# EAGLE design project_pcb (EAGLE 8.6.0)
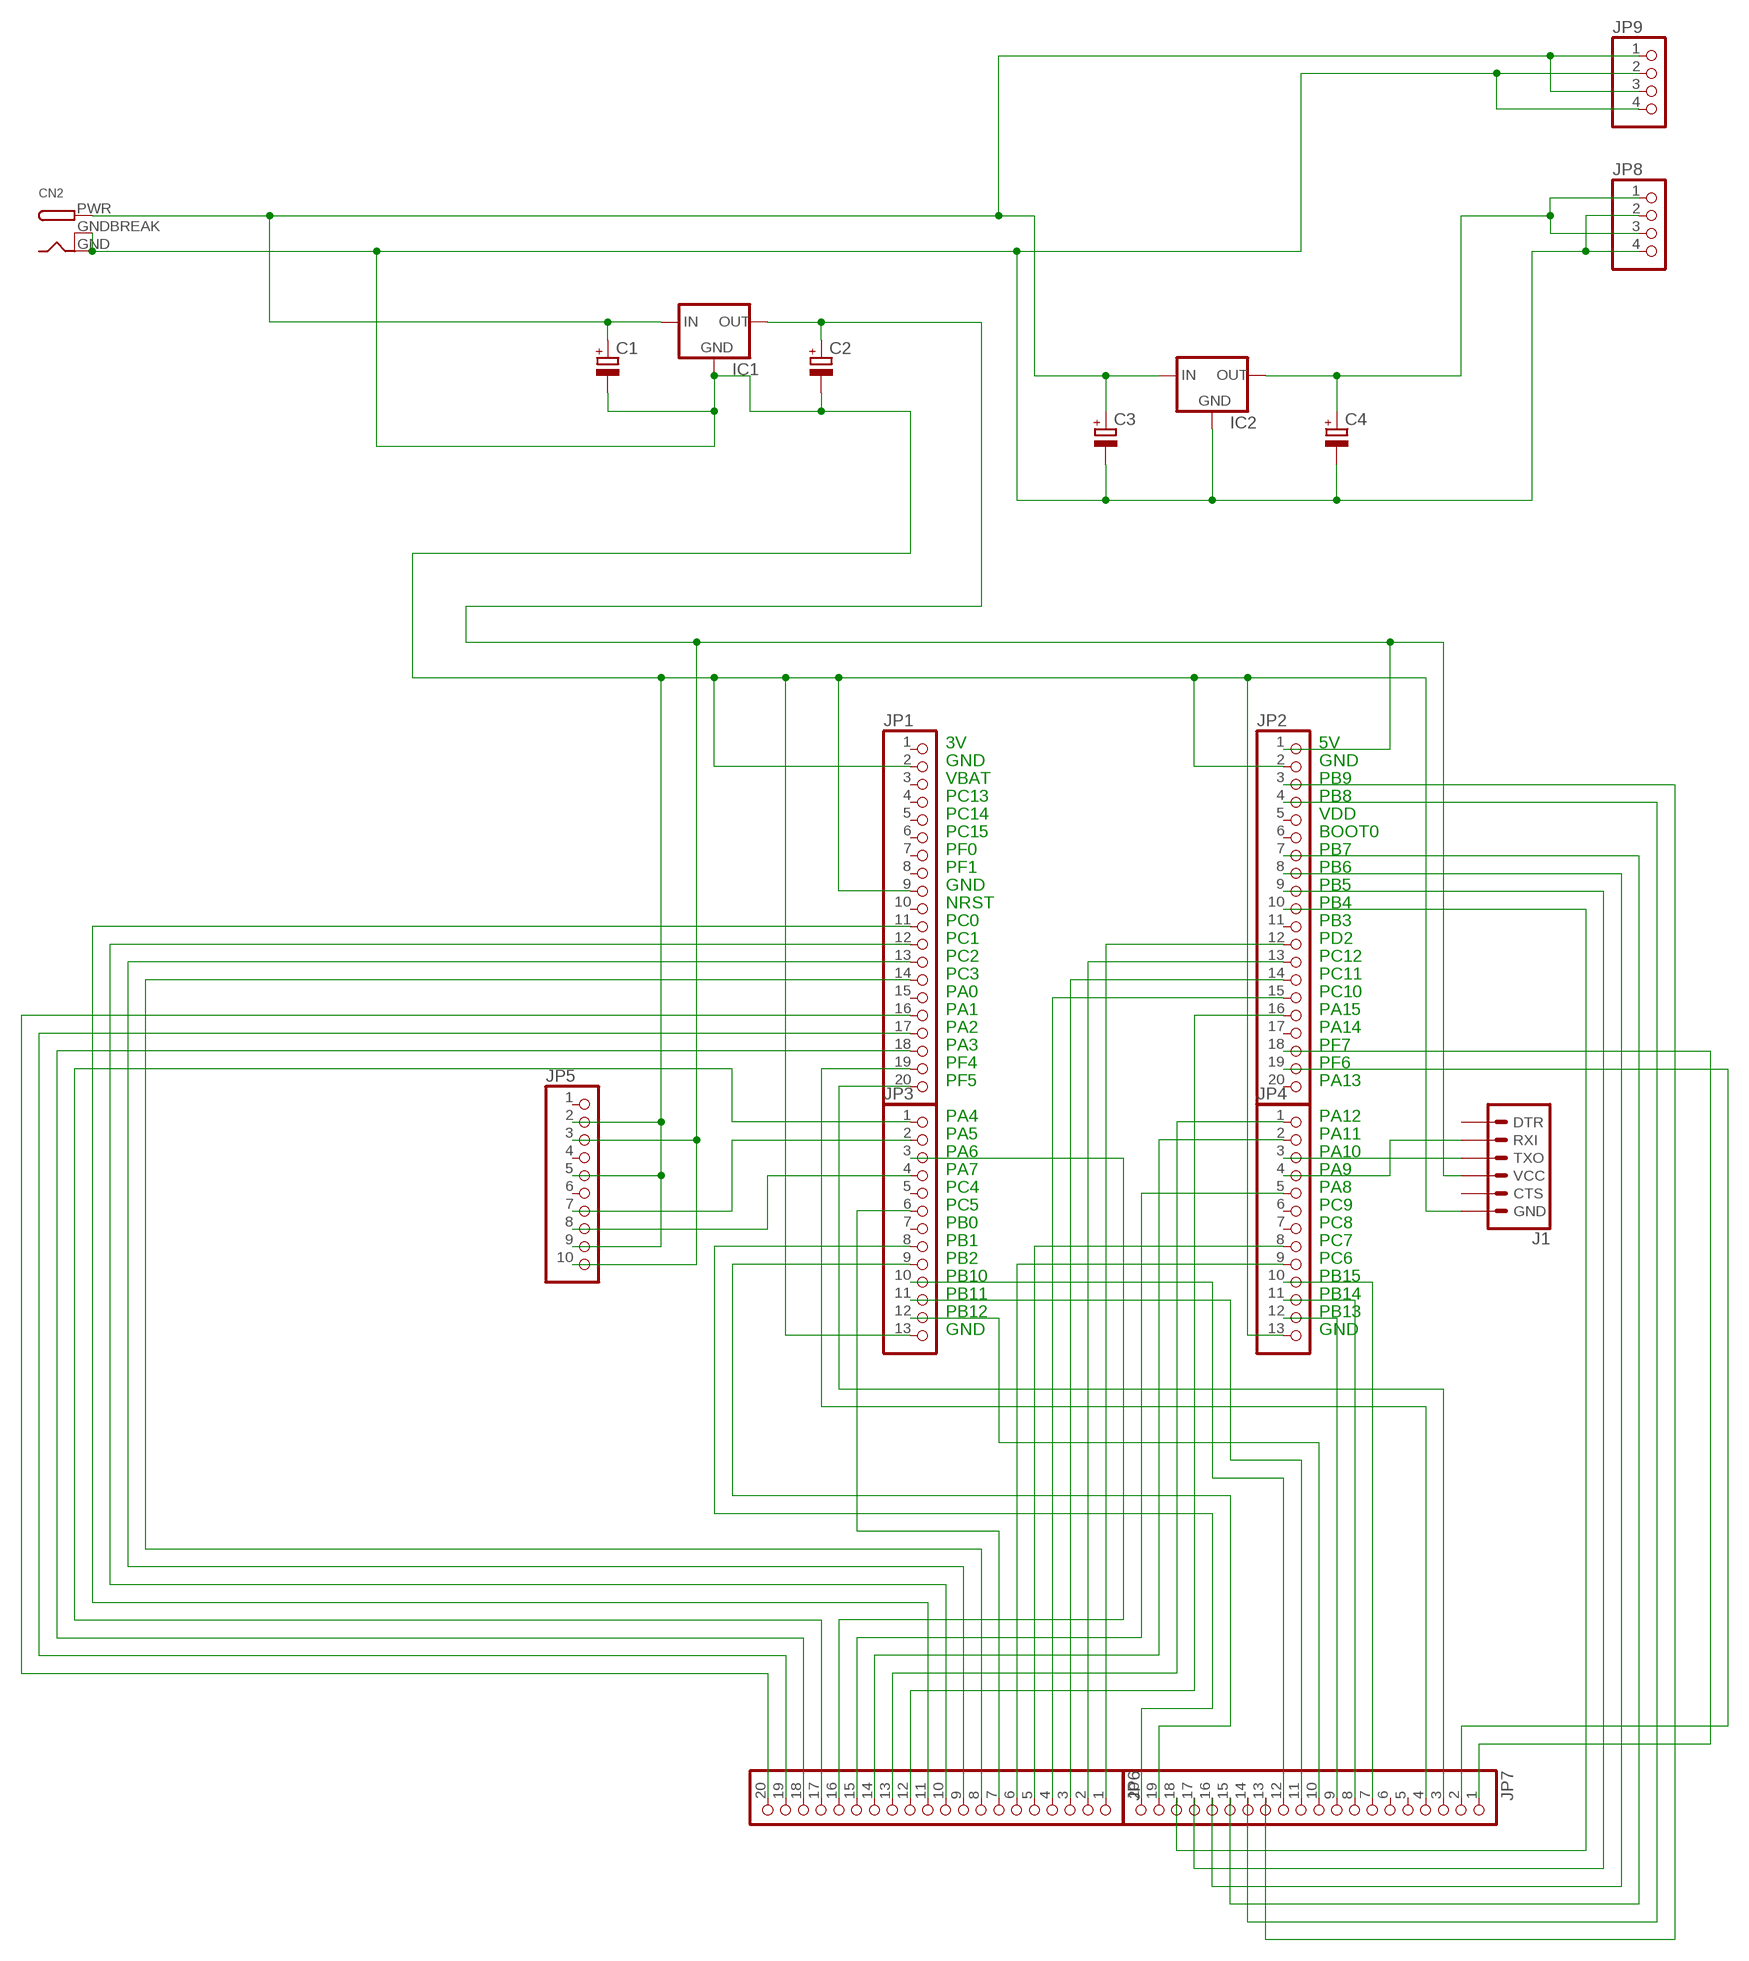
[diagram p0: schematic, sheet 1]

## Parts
C1  CPOL-EUE2.5-6  [E2,5-6]
C2  CPOL-EUE2.5-6  [E2,5-6]
C3  CPOL-EUE2.5-6  [E2,5-6]
C4  CPOL-EUE2.5-6  [E2,5-6]
CN2  DCBARRELPTH  [DCJACK_2MM_PTH]
IC1  78XXS  [78XXS]
IC2  78XXS  [78XXS]
J1  6_PIN_SERIAL_TARGET  [1X06]
JP1  PINHD-1X20  [1X20]
JP2  PINHD-1X20  [1X20]
JP3  PINHD-1X13  [1X13]
JP4  PINHD-1X13  [1X13]
JP5  PINHD-1X10  [1X10]
JP6  PINHD-1X20  [1X20]
JP7  PINHD-1X20  [1X20]
JP8  PINHD-1X4  [1X04]
JP9  PINHD-1X4  [1X04]

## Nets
N$1: J1.3(TXO) JP4.3
N$2: J1.2(RXI) JP4.4
N$3: C2.+ IC1.OUT J1.4(VCC) JP2.1 JP5.3 JP5.10
N$4: C1.- C2.- C3.- C4.- CN2.GND CN2.GNDBREAK IC1.GND IC2.GND J1.6(GND) JP1.2 JP1.9 JP2.2 JP3.13 JP4.13 JP5.2 JP5.5 JP5.9 JP8.2 JP8.4 JP9.2 JP9.4
N$5: JP3.2 JP5.7
N$6: JP3.4 JP5.8
N$7: JP1.16 JP6.20
N$8: JP1.17 JP6.19
N$9: JP1.18 JP6.18
N$10: JP3.1 JP6.17
N$11: JP3.3 JP6.16
N$12: JP4.5 JP6.15
N$13: JP4.2 JP6.14
N$14: JP4.1 JP6.13
N$15: JP2.16 JP6.12
N$16: JP1.11 JP6.11
N$17: JP1.12 JP6.10
N$18: JP1.13 JP6.9
N$19: JP1.14 JP6.8
N$20: JP3.6 JP6.7
N$21: JP4.9 JP6.6
N$22: JP4.8 JP6.5
N$23: JP2.15 JP6.4
N$24: JP2.14 JP6.3
N$25: JP2.13 JP6.2
N$26: JP2.10 JP7.18
N$27: JP3.8 JP7.20
N$28: JP3.9 JP7.19
N$29: JP2.9 JP7.17
N$30: JP2.8 JP7.16
N$31: JP2.7 JP7.15
N$32: JP2.4 JP7.14
N$33: JP2.3 JP7.13
N$34: JP3.10 JP7.12
N$35: JP3.11 JP7.11
N$36: JP3.12 JP7.10
N$37: JP4.12 JP7.9
N$38: JP4.11 JP7.8
N$39: JP4.10 JP7.7
N$40: JP2.18 JP7.1
N$41: JP2.19 JP7.2
N$42: JP1.20 JP7.3
N$43: JP1.19 JP7.4
N$44: JP2.12 JP6.1
N$45: C4.+ IC2.OUT JP8.1 JP8.3
N$47: C1.+ C3.+ CN2.PWR IC1.IN IC2.IN JP9.1 JP9.3
Unconnected: J1.1(DTR) J1.5(CTS) JP1.1 JP1.3 JP1.4 JP1.5 JP1.6 JP1.7 JP1.8 JP1.10 JP1.15 JP2.5 JP2.6 JP2.11 JP2.17 JP2.20 JP3.5 JP3.7 JP4.6 JP4.7 JP5.1 JP5.4 JP5.6 JP7.5 JP7.6

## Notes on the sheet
- 3V | 5V
- GND | GND
- VBAT | PB9
- PC13 | PB8
- PC14 | VDD
- PC15 | BOOT0
- PF0 | PB7
- PF1 | PB6
- GND | PB5
- NRST | PB4
- PC0 | PB3
- PC1 | PD2
- PC2 | PC12
- PC3 | PC11
- PA0 | PC10
- PA1 | PA15
- PA2 | PA14
- PA3 | PF7
- PF4 | PF6
- PF5 | PA13
- PA4 | PA12
- PA5 | PA11
- PA6 | PA10
- PA7 | PA9
- PC4 | PA8
- PC5 | PC9
- PB0 | PC8
- PB1 | PC7
- PB2 | PC6
- PB10 | PB15
- PB11 | PB14
- PB12 | PB13
- GND | GND

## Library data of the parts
C1-C4 = rcl:CPOL-EU: POLARIZED CAPACITOR, European symbol; SPICEPREFIX: C
CN2 = adafruit:DCBARREL: 2.0mm DC Barrel Jack DCJACK_2MM_PTH - Through Hole Jack (4UConnector: 05537)
IC1 IC2 = v-reg:78XXS: VOLTAGE REGULATOR
J1 = SparkFun-Connectors:6_PIN_SERIAL_TARGET: 6-pin header connection for use with the "FTDI BASIC" pinout - TARGET SIDE. Also known as "Arduino Serial Program Header". It is used to mate with our FTDI Basic serial programmers using the Arduino IDE. Note, this device has "TARGET" in the name. It is intended to be used on a design that contains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
JP1 JP2 JP6 JP7 = pinhead:PINHD-1X20: PIN HEADER
JP3 JP4 = pinhead:PINHD-1X13: PIN HEADER
JP5 = pinhead:PINHD-1X10: PIN HEADER
JP8 JP9 = pinhead:PINHD-1X4: PIN HEADER

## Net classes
0 default: width 0.305 mm

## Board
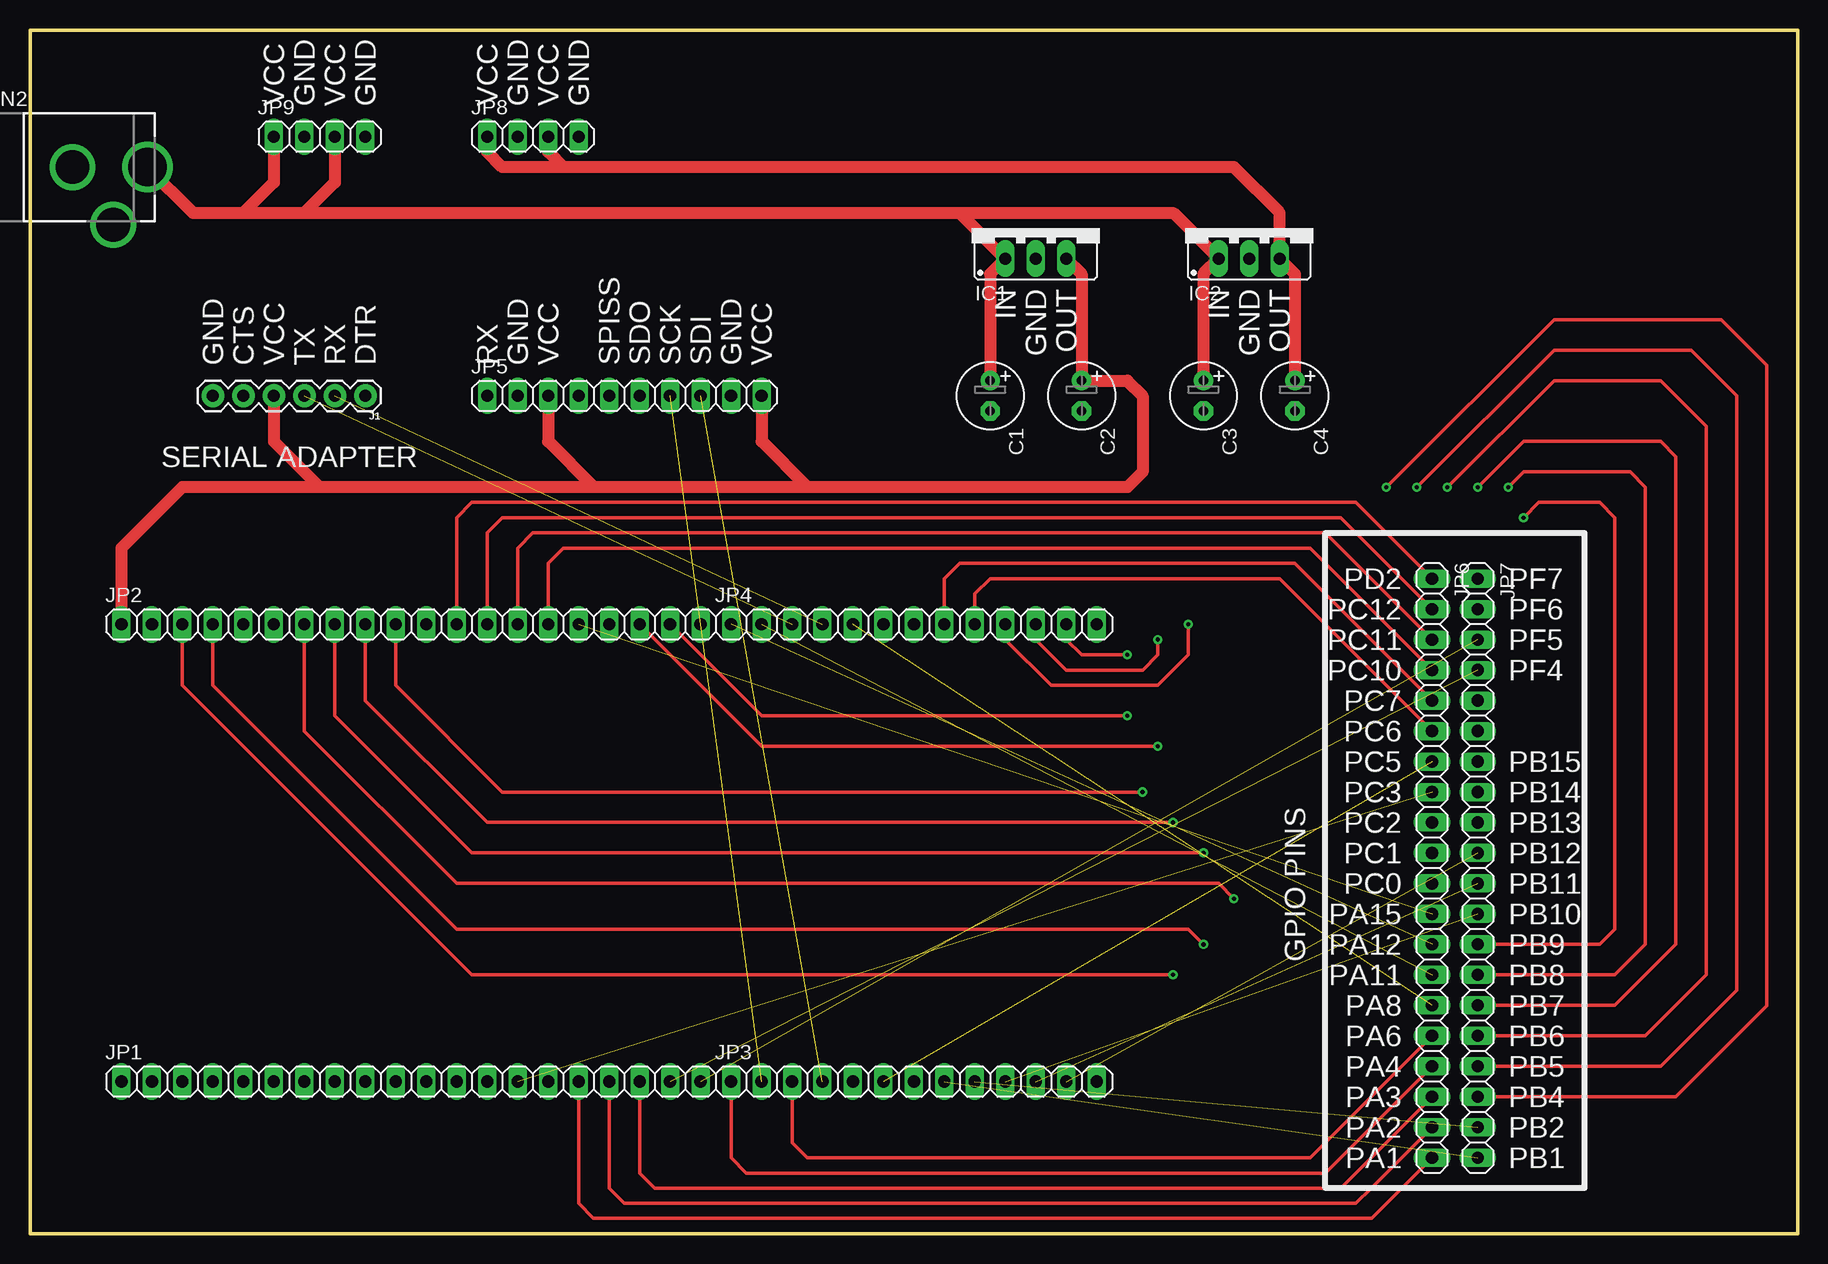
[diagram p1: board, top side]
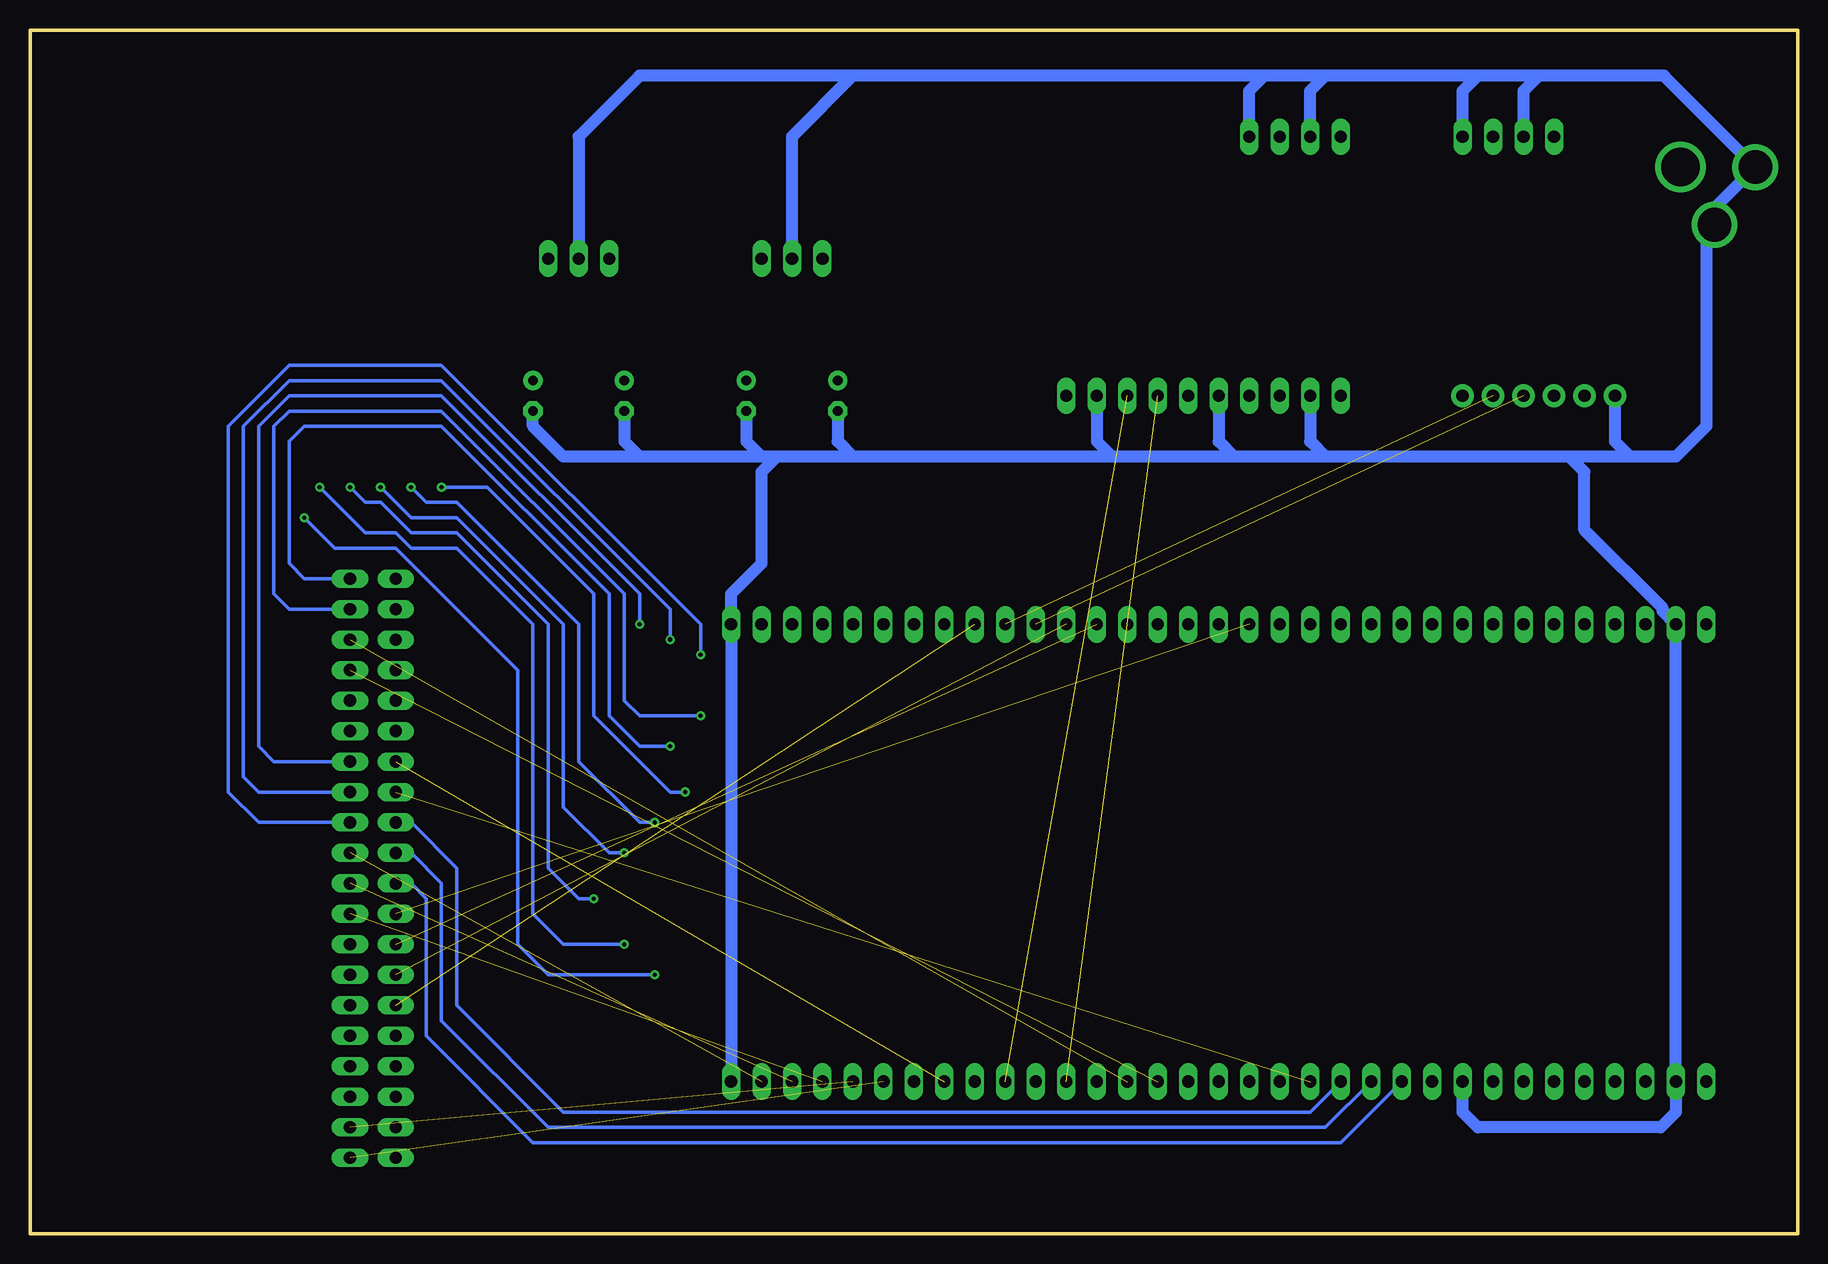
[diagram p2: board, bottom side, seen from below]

Size 147.32 x 100.33 mm. Coordinates in mm from the lower left corner, seen from the top.
Outline: 0,0 0,100.33 147.32,100.33 147.32,0 0,0
Copper layers (1*16): Top 0.035mm / dielectric 1.5mm / Bottom 0.035mm
Design rules "default": minimum track width 6mil, minimum drill 0.35mm, track to track 6mil, track to pad 6mil, pad to pad 6mil, via to via 6mil, smd to smd 6mil, copper to edge 40mil, drill to drill 6mil, minimum pad ring 10mil, minimum via ring 8mil, stop-mask expansion 4mil, vias tented up to drill 0mil, thermal gap 10mil

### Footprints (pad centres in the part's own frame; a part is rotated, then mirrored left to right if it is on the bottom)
E2,5-6 = drill 0.813 pad 1.6: + -1.27,0 | drill 0.813 pad 1.6 octagon: - 1.27,0
DCJACK_2MM_PTH = drill 2.8: GND 0,7.35; GNDBREAK 4.8,10.75 | drill 3.2: PWR 0,13.6
78XXS = drill 1.016 long: GND 0,-2.54; IN -2.54,-2.54; OUT 2.54,-2.54
1X06 = drill 1.016 pad 1.88: 1 0,0; 2 2.54,0; 3 5.08,0; 4 7.62,0; 5 10.16,0; 6 12.7,0
1X20 = drill 1.016 long: 1 -24.13,0; 2 -21.59,0; 3 -19.05,0; 4 -16.51,0; 5 -13.97,0; 6 -11.43,0; 7 -8.89,0; 8 -6.35,0; 9 -3.81,0; 10 -1.27,0; 11 1.27,0; 12 3.81,0; 13 6.35,0; 14 8.89,0; 15 11.43,0; 16 13.97,0; 17 16.51,0; 18 19.05,0; 19 21.59,0; 20 24.13,0
1X13 = drill 1.016 long: 1 -15.24,0; 2 -12.7,0; 3 -10.16,0; 4 -7.62,0; 5 -5.08,0; 6 -2.54,0; 7 0,0; 8 2.54,0; 9 5.08,0; 10 7.62,0; 11 10.16,0; 12 12.7,0; 13 15.24,0
1X10 = drill 1.016 long: 1 -11.43,0; 2 -8.89,0; 3 -6.35,0; 4 -3.81,0; 5 -1.27,0; 6 1.27,0; 7 3.81,0; 8 6.35,0; 9 8.89,0; 10 11.43,0
1X04 = drill 1.016 long: 1 -3.81,0; 2 -1.27,0; 3 1.27,0; 4 3.81,0

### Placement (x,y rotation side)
C1  80.01,69.85 270 top
C2  87.63,69.85 270 top
C3  97.79,69.85 270 top
C4  105.41,69.85 270 top
CN2  -3.81,88.9 270 top
IC1  83.82,83.82 0 top
IC2  101.6,83.82 0 top
J1  27.94,69.85 180 top
JP1  31.75,12.7 0 top
JP2  31.75,50.8 0 top
JP3  73.66,12.7 0 top
JP4  73.66,50.8 0 top
JP5  49.53,69.85 0 top
JP6  116.84,30.48 270 top
JP7  120.65,30.48 270 top
JP8  41.91,91.44 0 top
JP9  24.13,91.44 0 top

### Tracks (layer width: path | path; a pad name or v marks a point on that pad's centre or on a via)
N$1  (1 unrouted)
N$2  (1 unrouted)
N$3
  Top 1.016: IC1.OUT 87.63,80.01 C2.+ 91.44,71.12 92.71,69.85 92.71,63.5 91.44,62.23 64.77,62.23 | JP2.1 7.62,57.15 12.7,62.23 24.13,62.23 | 64.77,62.23 46.99,62.23 | 46.99,62.23 24.13,62.23 | J1.4 20.32,66.04 24.13,62.23 | JP5.3 43.18,66.04 46.99,62.23 | JP5.10 60.96,66.04 64.77,62.23
N$4
  Bottom 1.016: 21.59,96.52 11.16,96.52 CN2.GND 6.94,85.5 CN2.GNDBREAK 7.62,83.42 7.62,67.31 10.16,64.77 13.97,64.77 | 21.59,96.52 26.67,96.52 | 26.67,96.52 39.37,96.52 | 39.37,96.52 44.45,96.52 | 44.45,96.52 78.74,96.52 | 78.74,96.52 96.52,96.52 101.6,91.44 IC2.GND | IC1.GND 83.82,91.44 78.74,96.52 | 44.45,96.52 45.72,95.25 JP8.4 | JP8.2 40.64,95.25 39.37,96.52 | JP9.4 27.94,95.25 26.67,96.52 | JP9.2 22.86,95.25 21.59,96.52 | 13.97,64.77 19.05,64.77 | 19.05,64.77 39.37,64.77 | 39.37,64.77 46.99,64.77 | 46.99,64.77 57.15,64.77 | 57.15,64.77 78.74,64.77 | 78.74,64.77 85.09,64.77 | 85.09,64.77 86.36,64.77 | 86.36,64.77 96.52,64.77 | 96.52,64.77 102.87,64.77 105.41,67.31 C4.- | C3.- 97.79,66.04 96.52,64.77 | C2.- 87.63,66.04 86.36,64.77 | C1.- 80.01,66.04 78.74,64.77 | JP5.9 58.42,66.04 57.15,64.77 | JP5.5 48.26,66.04 46.99,64.77 | JP5.2 40.64,66.04 39.37,64.77 | J1.6 15.24,66.04 13.97,64.77 | 19.05,64.77 17.78,63.5 17.78,58.65 11.28,52.15 11.28,51.92 JP2.2 JP1.2 10.16,10.16 11.43,8.89 26.67,8.89 27.94,10.16 JP1.9 | 85.09,64.77 86.36,63.5 86.36,55.88 88.9,53.34 JP4.13 JP3.13
N$5  (1 unrouted)
N$6  (1 unrouted)
N$7
  Top 0.305: JP1.16 45.72,2.54 46.94,1.32 111.81,1.32 JP6.20
N$8
  Top 0.305: JP6.19 112.39,4.45 111.76,3.81 110.49,2.54 49.53,2.54 48.26,3.81 JP1.17
N$9
  Top 0.305: JP1.18 50.8,7.62 50.8,5.08 52.07,3.81 109.22,3.81 110.49,5.08 111.12,5.71 JP6.18
N$10
  Top 0.305: JP3.1 58.42,6.35 59.69,5.08 107.95,5.08 JP6.17
N$11
  Top 0.305: JP3.3 63.5,7.62 64.77,6.35 106.68,6.35 JP6.16
N$12  (1 unrouted)
N$13  (1 unrouted)
N$14  (1 unrouted)
N$15  (1 unrouted)
N$16
  Bottom 0.305: JP6.11 115.57,29.21 114.3,27.94 114.3,16.51 105.41,7.62 38.1,7.62 JP1.11
N$17
  Bottom 0.305: JP6.10 115.57,31.75 113.03,29.21 113.03,17.78 104.14,8.89 39.37,8.89 JP1.12
N$18
  Bottom 0.305: JP1.13 40.64,10.16 102.87,10.16 111.76,19.05 111.76,30.48 115.57,34.29 JP6.9
N$19  (1 unrouted)
N$20  (1 unrouted)
N$21
  Top 0.305: JP6.6 104.14,54.61 80.01,54.61 78.74,53.34 JP4.9
N$22
  Top 0.305: JP6.5 105.41,55.88 77.47,55.88 76.2,54.61 JP4.8
N$23
  Top 0.305: JP6.4 106.68,57.15 44.45,57.15 43.18,55.88 JP2.15
N$24
  Top 0.305: JP6.3 107.95,58.42 41.91,58.42 40.64,57.15 JP2.14
N$25
  Top 0.305: 116.84,52.34 JP6.2 109.22,59.69 39.37,59.69 38.1,58.42 JP2.13
N$26  (via drill 0.35)
  Top 0.305: JP7.18 137.16,11.43 144.73,19 144.73,72.39 140.92,76.2 127,76.2 v113.03,62.23 | JP2.10 30.48,45.72 39.37,36.83 v92.71,36.83
  Bottom 0.305: v113.03,62.23 109.22,62.23 100.33,53.34 100.33,43.18 93.98,36.83 v92.71,36.83
N$27  (1 unrouted)
N$28  (1 unrouted)
N$29  (via drill 0.35)
  Top 0.305: JP7.17 135.89,13.97 142.24,20.32 142.24,69.85 138.43,73.66 127,73.66 v115.57,62.23 | v95.25,34.29 38.1,34.29 27.94,44.45 JP2.9
  Bottom 0.305: v115.57,62.23 114.3,60.96 111.76,60.96 101.6,50.8 101.6,39.37 96.52,34.29 v95.25,34.29
N$30  (via drill 0.35)
  Top 0.305: JP7.16 134.62,16.51 139.7,21.59 139.7,67.31 135.89,71.12 127,71.12 v118.11,62.23 | JP2.8 25.4,43.18 36.83,31.75 v97.79,31.75
  Bottom 0.305: v118.11,62.23 115.57,59.69 111.76,59.69 102.87,50.8 102.87,35.56 99.06,31.75 v97.79,31.75
N$31  (via drill 0.35)
  Top 0.305: JP7.15 132.08,19.05 137.16,24.13 137.16,64.77 135.89,66.04 124.46,66.04 v120.65,62.23 | v100.33,27.94 99.06,29.21 35.56,29.21 22.86,41.91 JP2.7
  Bottom 0.305: v120.65,62.23 119.38,60.96 118.11,60.96 115.57,58.42 111.76,58.42 104.14,50.8 104.14,30.48 101.6,27.94 v100.33,27.94
N$32  (via drill 0.35)
  Top 0.305: JP7.14 132.08,21.59 134.62,24.13 134.62,62.23 133.35,63.5 124.46,63.5 v123.19,62.23 | v97.79,24.13 96.52,25.4 35.56,25.4 15.24,45.72 JP2.4
  Bottom 0.305: v123.19,62.23 119.38,58.42 116.84,58.42 115.57,57.15 111.76,57.15 105.41,50.8 105.41,26.67 102.87,24.13 v97.79,24.13
N$33  (via drill 0.35)
  Top 0.305: JP7.13 130.81,24.13 132.08,25.4 132.08,59.69 130.81,60.96 125.73,60.96 v124.46,59.69 | v95.25,21.59 36.83,21.59 12.7,45.72 JP2.3
  Bottom 0.305: v124.46,59.69 121.92,57.15 116.84,57.15 106.68,46.99 106.68,24.13 104.14,21.59 v95.25,21.59
N$34  (1 unrouted)
N$35  (1 unrouted)
N$36  (1 unrouted)
N$37  (via drill 0.35)
  Top 0.305: v91.44,48.26 87.63,48.26 86.36,49.53 JP4.12
  Bottom 0.305: JP7.9 128.27,34.29 130.81,36.83 130.81,67.31 125.73,72.39 113.03,72.39 91.44,50.8 v91.44,48.26
N$38  (via drill 0.35)
  Top 0.305: JP4.11 83.82,49.53 86.36,46.99 92.71,46.99 93.98,48.26 v93.98,49.53
  Bottom 0.305: JP7.8 128.27,36.83 129.54,38.1 129.54,67.31 125.73,71.12 113.03,71.12 93.98,52.07 v93.98,49.53
N$39  (via drill 0.35)
  Top 0.305: JP4.10 81.28,49.53 85.09,45.72 93.98,45.72 96.52,48.26 v96.52,50.8
  Bottom 0.305: JP7.7 127,39.37 128.27,40.64 128.27,67.31 125.73,69.85 113.03,69.85 96.52,53.34 v96.52,50.8
N$40  (via drill 0.35)
  Top 0.305: v93.98,40.64 60.96,40.64 JP2.18
  Bottom 0.305: JP7.1 124.46,54.61 125.73,55.88 125.73,66.04 124.46,67.31 113.03,67.31 99.06,53.34 99.06,43.18 96.52,40.64 v93.98,40.64
N$41  (via drill 0.35)
  Top 0.305: v91.44,43.18 60.96,43.18 JP2.19
  Bottom 0.305: JP7.2 125.73,52.07 127,53.34 127,67.31 125.73,68.58 113.03,68.58 97.79,53.34 97.79,44.45 96.52,43.18 v91.44,43.18
N$42  (1 unrouted)
N$43  (1 unrouted)
N$44
  Top 0.305: JP6.1 110.49,60.96 36.83,60.96 35.56,59.69 JP2.12
N$45
  Top 1.016: C4.+ 105.41,80.01 IC2.OUT 104.14,85.09 100.33,88.9 44.45,88.9 | 44.45,88.9 39.37,88.9 38.1,90.17 JP8.1 | JP8.3 43.18,90.17 44.45,88.9
N$47
  Top 1.016: CN2.PWR 13.6,85.09 17.78,85.09 | 17.78,85.09 22.86,85.09 | 22.86,85.09 77.47,85.09 | 77.47,85.09 95.25,85.09 IC2.IN 97.79,80.01 C3.+ | 77.47,85.09 IC1.IN 80.01,80.01 C1.+ | JP9.1 20.32,87.63 17.78,85.09 | JP9.3 25.4,87.63 22.86,85.09

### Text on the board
tPlace: VCC | GND | VCC | GND | VCC | GND | VCC | GND | IN | GND | OUT | IN | GND | OUT | GND | CTS | VCC | TX | RX | DTR | RX | GND | VCC | SPISS | SDO | SCK | SDI | GND | VCC | SERIAL ADAPTER | PD2 | PF7 | PC12 | PF6 | PC11 | PF5 | PC10 | PF4 | PC7 | PC6 | PC5 | PB15 | PC3 | PB14 | GPIO PINS | PC2 | PB13 | PC1 | PB12 | PC0 | PB11 | PA15 | PB10 | PA12 | PB9 | PA11 | PB8 | PA8 | PB7 | PA6 | PB6 | PA4 | PB5 | PA3 | PB4 | PA2 | PB2 | PA1 | PB1

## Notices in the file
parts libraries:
SparkFun-Connectors: Licensing: Creative Commons ShareAlike 4.0 International - https://creativecommons.org/licenses/by-sa/4.0
